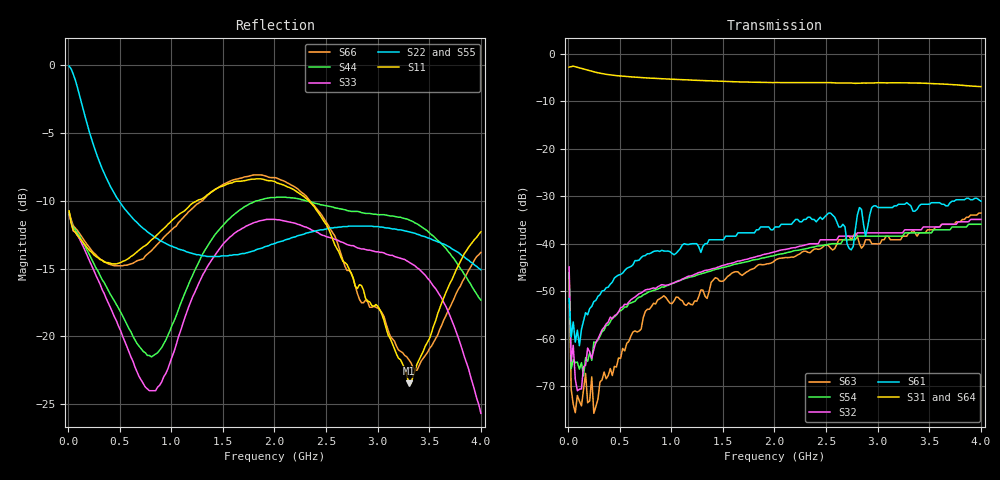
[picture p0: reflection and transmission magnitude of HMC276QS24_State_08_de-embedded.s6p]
! Hittite Microwave Corporation
! 20 Alpha Road
! Chelmsford, MA 01824
! Tel: 978-250-3343
! Fax: 978-250-3373
! Device: HMC276QS24, 0.7-3.0 GHz, GaAS MMIC 4x2 Switch Matrix in 24-lead QSOP package
! Misc: Data was de-embedded to package pins.
!  Port 1 = OP1
!  Port 2 = VL
!  Port 3 = VH
!  Port 4 = HH
!  Port 5 = HL
!  Port 6 = OP2
!  Vdd = +5 V
!  Vctl = 0 V[Logic 0] / +5 V[Logic 1]
!  State 08,  VH to OP1,  HH to OP2
!  Control Lines (Logic)
!  HV 1 = 0, Tone 1 = 1
!  HV 2 = 1, Tone 2 = 1
!  Data reformated to new Touchstone file format - Wed Jan 10 14:36:49 2007
# MHz S DB R 50
! 6 Port Network Data
! Created Wed Jan 10 15:18:00 2007
! # mhz S db R 50
! 6 Port Network Data from SP1.SP block
! freq  dbS11  angS11  dbS12  angS12  dbS13  angS13  dbS14  angS14
!  dbS15  angS15  dbS16  angS16
!  dbS21  angS21  dbS22  angS22
!  dbS23  angS23  dbS24  angS24  dbS25  angS25  dbS26  angS26
!  dbS31  angS31  dbS32  angS32  dbS33  angS33  dbS34  angS34
!  dbS35  angS35  dbS36  angS36
!  dbS41  angS41  dbS42  angS42
!  dbS43  angS43  dbS44  angS44  dbS45  angS45  dbS46  angS46
!  dbS51  angS51  dbS52  angS52  dbS53  angS53  dbS54  angS54
!  dbS55  angS55  dbS56  angS56
!  dbS61  angS61  dbS62  angS62
!  dbS63  angS63  dbS64  angS64  dbS65  angS65  dbS66  angS66
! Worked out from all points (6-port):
!   201 points, 10 MHz to 4 GHz, reference 50 ohm
!   strongest paths, dB at 10 MHz, 1.008 GHz, 2.005 GHz, 3.002 GHz, 4 GHz:
!     S31: -2.9, -5.4, -6.1, -6.1, -7.0
!     S64: -2.9, -5.4, -6.2, -6.3, -7.0
!     S61: -51.5, -42.1, -36.5, -32.4, -31.1
!     S32: -44.9, -48.4, -41.7, -37.7, -34.9
!     S54: -46.2, -48.4, -42.4, -38.4, -35.9
!     S63: -46.4, -52.6, -43.5, -40.1, -33.6
!   lowest |S11| = -23.5 dB at 3.302 GHz (marker M1), VSWR 1.14, Z = 56.3 + j3.37 ohm
!   |S11| at or under -10 dB: start of sweep to 1.248 GHz; 2.333 GHz to end of sweep
